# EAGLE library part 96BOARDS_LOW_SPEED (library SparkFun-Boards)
96 BOARDS SPEC LOW SPEED CONNECTOR 2x20, 40-pin, header for low speed expansion. Has UARTS, I2C, I2S, SPI and GPIO. * 2mm-pitch variant interfaces directly with the header on a 96-boards-compliant board. * 0.1-pitch version is for applications where the header has been translated to the larger, more available 0.1" 2x20 connector. For more details, see the spec at https://www.96boards.org
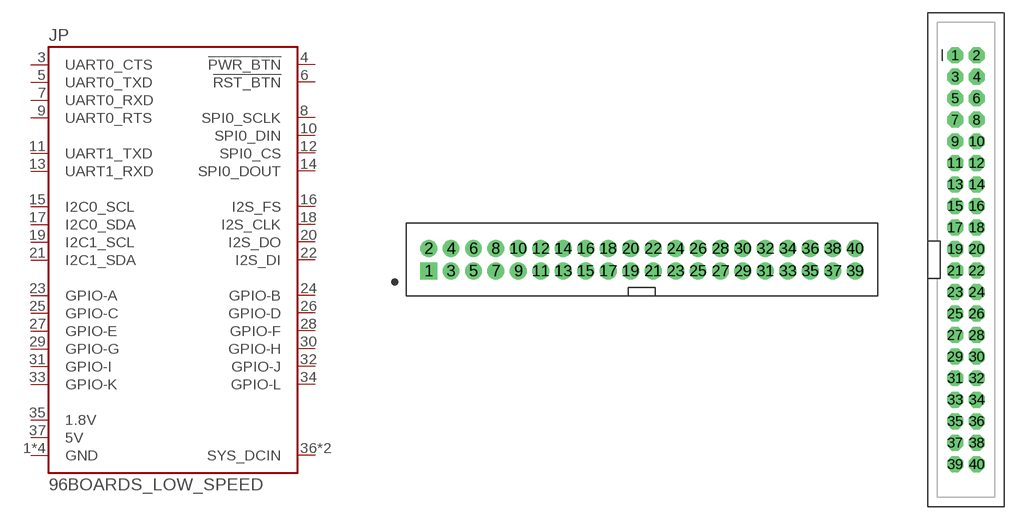
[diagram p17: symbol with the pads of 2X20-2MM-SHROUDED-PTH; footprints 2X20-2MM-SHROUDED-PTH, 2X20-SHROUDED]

Designator prefix JP

## 96BOARDS_LOW_SPEEDPTH  [2X20-2MM-SHROUDED-PTH]
1  GND  pwr
2  GND  pwr
3  UART0_CTS  out
4  !PWR_BTN
5  UART0_TXD  out
6  !RST_BTN
7  UART0_RXD  in
8  SPI0_SCLK  out
9  UART0_RTS  in
10  SPI0_DIN  in
11  UART1_TXD  out
12  SPI0_CS  out
13  UART1_RXD  in
14  SPI0_DOUT  out
15  I2C0_SCL
16  I2S_FS
17  I2C0_SDA
18  I2S_CLK
19  I2C1_SCL
20  I2S_DO
21  I2C1_SDA
22  I2S_DI
23  GPIO-A
24  GPIO-B
25  GPIO-C
26  GPIO-D
27  GPIO-E
28  GPIO-F
29  GPIO-G
30  GPIO-H
31  GPIO-I
32  GPIO-J
33  GPIO-K
34  GPIO-L
35  1.8V  pwr
36  SYS_DCIN  pwr
37  5V  pwr
38  SYS_DCIN  pwr
39  GND  pwr
40  GND  pwr

## 96BOARDS_LOW_SPEED0.1"-PTH  [2X20-SHROUDED]
Pads as for 2X20-2MM-SHROUDED-PTH

## 96BOARDS_LOW_SPEEDSMT-F (PROD_ID: CONN-12977)  [2X20-2MM-SMT-F]
Pads as for 2X20-2MM-SHROUDED-PTH

## 96BOARDS_LOW_SPEEDSMT-M-BOTTOM (PROD_ID: CONN-12975)  [2X20-2MM-SHROUDED-SMT-BOTTOM-M]
Pads as for 2X20-2MM-SHROUDED-PTH

## 96BOARDS_LOW_SPEED  [2X20-2MM-SHROUDED-RA-PTH]
Pads as for 2X20-2MM-SHROUDED-PTH

## 96BOARDS_LOW_SPEEDSMT-M-TOP (PROD_ID: CONN-12975)  [2X20-2MM-SHROUDED-SMT-TOP-M]
Pads as for 2X20-2MM-SHROUDED-PTH

## 96BOARDS_LOW_SPEEDRIBBON-COMPATIBLE  [2X20-2MM-SHROUDED-SMT-RIBBON-M]
Pads as for 2X20-2MM-SHROUDED-PTH

## Footprint 2X20-2MM-SHROUDED-PTH (pad centres in mm)
drill 1 square: 1 -19,-1
drill 1: 2 -19,1; 3 -17,-1; 4 -17,1; 5 -15,-1; 6 -15,1; 7 -13,-1; 8 -13,1; 9 -11,-1; 10 -11,1; 11 -9,-1; 12 -9,1; 13 -7,-1; 14 -7,1; 15 -5,-1; 16 -5,1; 17 -3,-1; 18 -3,1; 19 -1,-1; 20 -1,1; 21 1,-1; 22 1,1; 23 3,-1; 24 3,1; 25 5,-1; 26 5,1; 27 7,-1; 28 7,1; 29 9,-1; 30 9,1; 31 11,-1; 32 11,1; 33 13,-1; 34 13,1; 35 15,-1; 36 15,1; 37 17,-1; 38 17,1; 39 19,-1; 40 19,1

## Footprint 2X20-SHROUDED (pad centres in mm)
drill 1.016 pad 1.88 octagon: 1 -1.27,24.13; 2 1.27,24.13; 3 -1.27,21.59; 4 1.27,21.59; 5 -1.27,19.05; 6 1.27,19.05; 7 -1.27,16.51; 8 1.27,16.51; 9 -1.27,13.97; 10 1.27,13.97; 11 -1.27,11.43; 12 1.27,11.43; 13 -1.27,8.89; 14 1.27,8.89; 15 -1.27,6.35; 16 1.27,6.35; 17 -1.27,3.81; 18 1.27,3.81; 19 -1.27,1.27; 20 1.27,1.27; 21 -1.27,-1.27; 22 1.27,-1.27; 23 -1.27,-3.81; 24 1.27,-3.81; 25 -1.27,-6.35; 26 1.27,-6.35; 27 -1.27,-8.89; 28 1.27,-8.89; 29 -1.27,-11.43; 30 1.27,-11.43; 31 -1.27,-13.97; 32 1.27,-13.97; 33 -1.27,-16.51; 34 1.27,-16.51; 35 -1.27,-19.05; 36 1.27,-19.05; 37 -1.27,-21.59; 38 1.27,-21.59; 39 -1.27,-24.13; 40 1.27,-24.13

## Footprint 2X20-2MM-SMT-F (pad centres in mm)
E.G. Molex 87832-4072
smd 0.8 x 1.5: 1 -19,-2.75; 2 -19,2.75; 3 -17,-2.75; 4 -17,2.75; 5 -15,-2.75; 6 -15,2.75; 7 -13,-2.75; 8 -13,2.75; 9 -11,-2.75; 10 -11,2.75; 11 -9,-2.75; 12 -9,2.75; 13 -7,-2.75; 14 -7,2.75; 15 -5,-2.75; 16 -5,2.75; 17 -3,-2.75; 18 -3,2.75; 19 -1,-2.75; 20 -1,2.75; 21 1,-2.75; 22 1,2.75; 23 3,-2.75; 24 3,2.75; 25 5,-2.75; 26 5,2.75; 27 7,-2.75; 28 7,2.75; 29 9,-2.75; 30 9,2.75; 31 11,-2.75; 32 11,2.75; 33 13,-2.75; 34 13,2.75; 35 15,-2.75; 36 15,2.75; 37 17,-2.75; 38 17,2.75; 39 19,-2.75; 40 19,2.75
hole 0.8 at -20,0
hole 0.8 at 20,0

## Footprint 2X20-2MM-SHROUDED-SMT-BOTTOM-M (pad centres in mm)
Warning! this is for the BOTTOM of a 96-boards Layout Pin 1 is not in the right place for ordinary usage!! Candidate parts: Molex 87832-4072 - shrouded Molex 87759-4050 - unshrouded
smd 1 x 2.75: 1 19,-2.125; 2 19,2.125; 3 17,-2.125; 4 17,2.125; 5 15,-2.125; 6 15,2.125; 7 13,-2.125; 8 13,2.125; 9 11,-2.125; 10 11,2.125; 11 9,-2.125; 12 9,2.125; 13 7,-2.125; 14 7,2.125; 15 5,-2.125; 16 5,2.125; 17 3,-2.125; 18 3,2.125; 19 1,-2.125; 20 1,2.125; 21 -1,-2.125; 22 -1,2.125; 23 -3,-2.125; 24 -3,2.125; 25 -5,-2.125; 26 -5,2.125; 27 -7,-2.125; 28 -7,2.125; 29 -9,-2.125; 30 -9,2.125; 31 -11,-2.125; 32 -11,2.125; 33 -13,-2.125; 34 -13,2.125; 35 -15,-2.125; 36 -15,2.125; 37 -17,-2.125; 38 -17,2.125; 39 -19,-2.125; 40 -19,2.125
hole 0.8 at -18,0
hole 0.8 at 18,0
